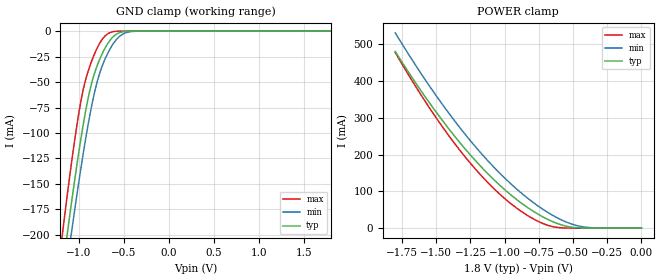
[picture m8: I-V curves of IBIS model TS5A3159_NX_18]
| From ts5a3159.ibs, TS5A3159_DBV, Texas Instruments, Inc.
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[Model]   TS5A3159_NX_18
Model_type  Terminator
| variable   typ   min   max
C_comp   25.08pF   23.19pF   25.88pF
| C_tri-state   25.08pF   23.19pF   25.88pF
[Temperature Range]   40   100   -40
| Ambient temperature   25   85   -40
[Voltage range]   1.8   1.65   1.95
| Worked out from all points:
|   GND clamp passes 1 mA (typ) near -0.53 V on its own axis
|   POWER clamp passes 1 mA (typ) near -0.46 V on its own axis
[GND Clamp]
| TS5A3159_NX_18
|   Voltage   I(typ)   I(min)   I(max)
-1.8V     -727.5mA   -735.4mA   -727mA
-1.175V   -233.4mA   -261.3mA   -196.8mA
-1.115V   -192.8mA   -221.6mA   -154.4mA
-1.08V    -170mA     -199.2mA   -131mA
-990mV    -115.1mA   -144.3mA   -77.15mA
-915mV    -75.64mA   -102.7mA   -45.85mA
-855mV    -51.29mA   -73.69mA   -29.63mA
-800mV    -35.56mA   -52.09mA   -17.9mA
-675mV    -12.08mA   -21.59mA   -2.59mA
-535mV    -1.209mA   -4.477mA   -47.67uA
-390mV    -28.86uA   -271.3uA   -169nA
1.8V      594.9pA    7.561uA    39.07pA
[POWER Clamp]
| TS5A3159_NX_18
|   Voltage   I(typ)   I(min)   I(max)
-1.8V     479.7mA    530.3mA    477.1mA
-1.555V   343mA      388.8mA    329.5mA
-1.325V   231.1mA    271.7mA    210.3mA
-1.105V   141.1mA    175.9mA    117mA
-1V       104.7mA    136.2mA    80.53mA
-895mV    72.84mA    100.6mA    49.83mA
-785mV    44.55mA    68.02mA    24.22mA
-690mV    24.74mA    43.94mA    8.374mA
-590mV    9.47mA     23.32mA    1.099mA
-495mV    2.004mA    9.442mA    61.98uA
-355mV    65.8uA     963.5uA    300.2nA
0V        0A         0A         0A
